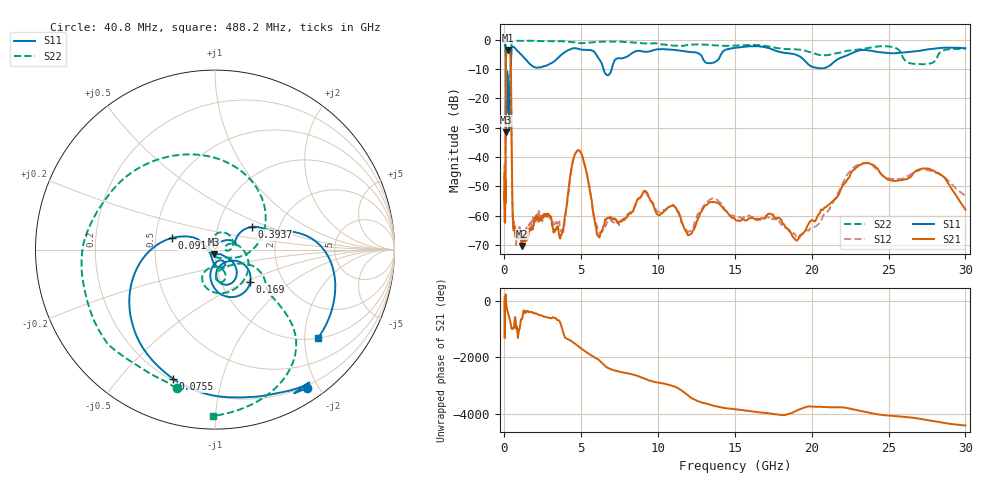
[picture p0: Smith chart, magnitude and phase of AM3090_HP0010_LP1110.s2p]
! Date/Time: Thu, Feb 28, 2019 1:55 PM
! Network Analyzer: Agilent Technologies E8364B Rev: A.07.50.67
! Sweep from 0.010 to 30.000 GHz, 1601 Points, Sweep Type: LOG
! Power Supply: 5.023 V, 0.002 A
# Hz S DB R 50
!freq MagS11 AngS11 MagS21 AngS21 MagS12 AngS12 MagS22 AngS22
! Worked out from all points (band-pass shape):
!   1601 points, 10 MHz to 30 GHz, reference 50 ohm
!   highest |S21| = -3.43 dB at 253.4 MHz (marker M1); lowest = -70.4 dB at 1.115 GHz (marker M2)
!   |S21| within 3 dB of the highest: 103 MHz to 396.5 MHz (293.5 MHz wide, 118 % of centre)
!   lowest |S11| = -31.6 dB at 99.92 MHz (marker M3), VSWR 1.05, Z = 49.5 - j2.57 ohm
!   |S11| at or under -10 dB: 90.67 MHz to 409.1 MHz (318.4 MHz wide, 127 % of centre); 6.451 GHz to 6.98 GHz (529.1 MHz wide, 7.88 % of centre)
!   |S22| runs from -33.3 to -0.2 dB; largest |S21 - S12| = 0.013
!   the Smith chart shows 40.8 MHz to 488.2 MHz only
!   S11 on the Smith chart (normalised r, x): 40.8 MHz: 0.17, -1.86; 75.5 MHz: 0.21, -0.71; 91.78 MHz: 0.61, +0.08; 169 MHz: 1.37, -0.54; 393.7 MHz: 1.45, +0.39; 488.2 MHz: 1.01, -2.33
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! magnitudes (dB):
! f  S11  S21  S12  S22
! 10 MHz  -0.2  -62.0  -44.5  -0.6
! 11.05 MHz  -0.5  -45.4  -43.1  -1.0
! 38.04 MHz  -0.5  -61.5  -60.8  -1.7
! 40.8 MHz  -0.7  -60.0  -61.3  -1.9
! 75.5 MHz  -2.4  -48.1  -46.2  -4.4
! 91.78 MHz  -12.0  -14.7  -14.6  -12.9
! 99.92 MHz  -31.6  -7.4  -7.4  -32.9
! 144.7 MHz  -19.5  -3.7  -3.6  -24.2
! 169 MHz  -11.5  -3.5  -3.5  -14.5
! 253.4 MHz  -22.6  -3.4  -3.4  -17.4
! 393.7 MHz  -12.4  -6.2  -6.2  -10.3
! 488.2 MHz  -2.4  -44.4  -44.5  -0.7
! 550.5 MHz  -2.3  -61.5  -60.2  -0.4
! 1.115 GHz  -5.1  -70.4  -67.3  -0.3
! 2.084 GHz  -9.5  -60.9  -61.0  -0.3
! 3.686 GHz  -5.2  -66.5  -65.2  -0.4
! 4.805 GHz  -3.1  -37.7  -37.6  -1.1
! 6.11 GHz  -6.2  -67.1  -65.6  -0.6
! 7.926 GHz  -5.9  -60.8  -60.9  -0.7
! 19.31 GHz  -6.0  -66.5  -66.6  -3.4
! 23.48 GHz  -3.5  -42.1  -42.1  -3.0
! 30 GHz  -2.8  -58.0  -53.3  -3.0
